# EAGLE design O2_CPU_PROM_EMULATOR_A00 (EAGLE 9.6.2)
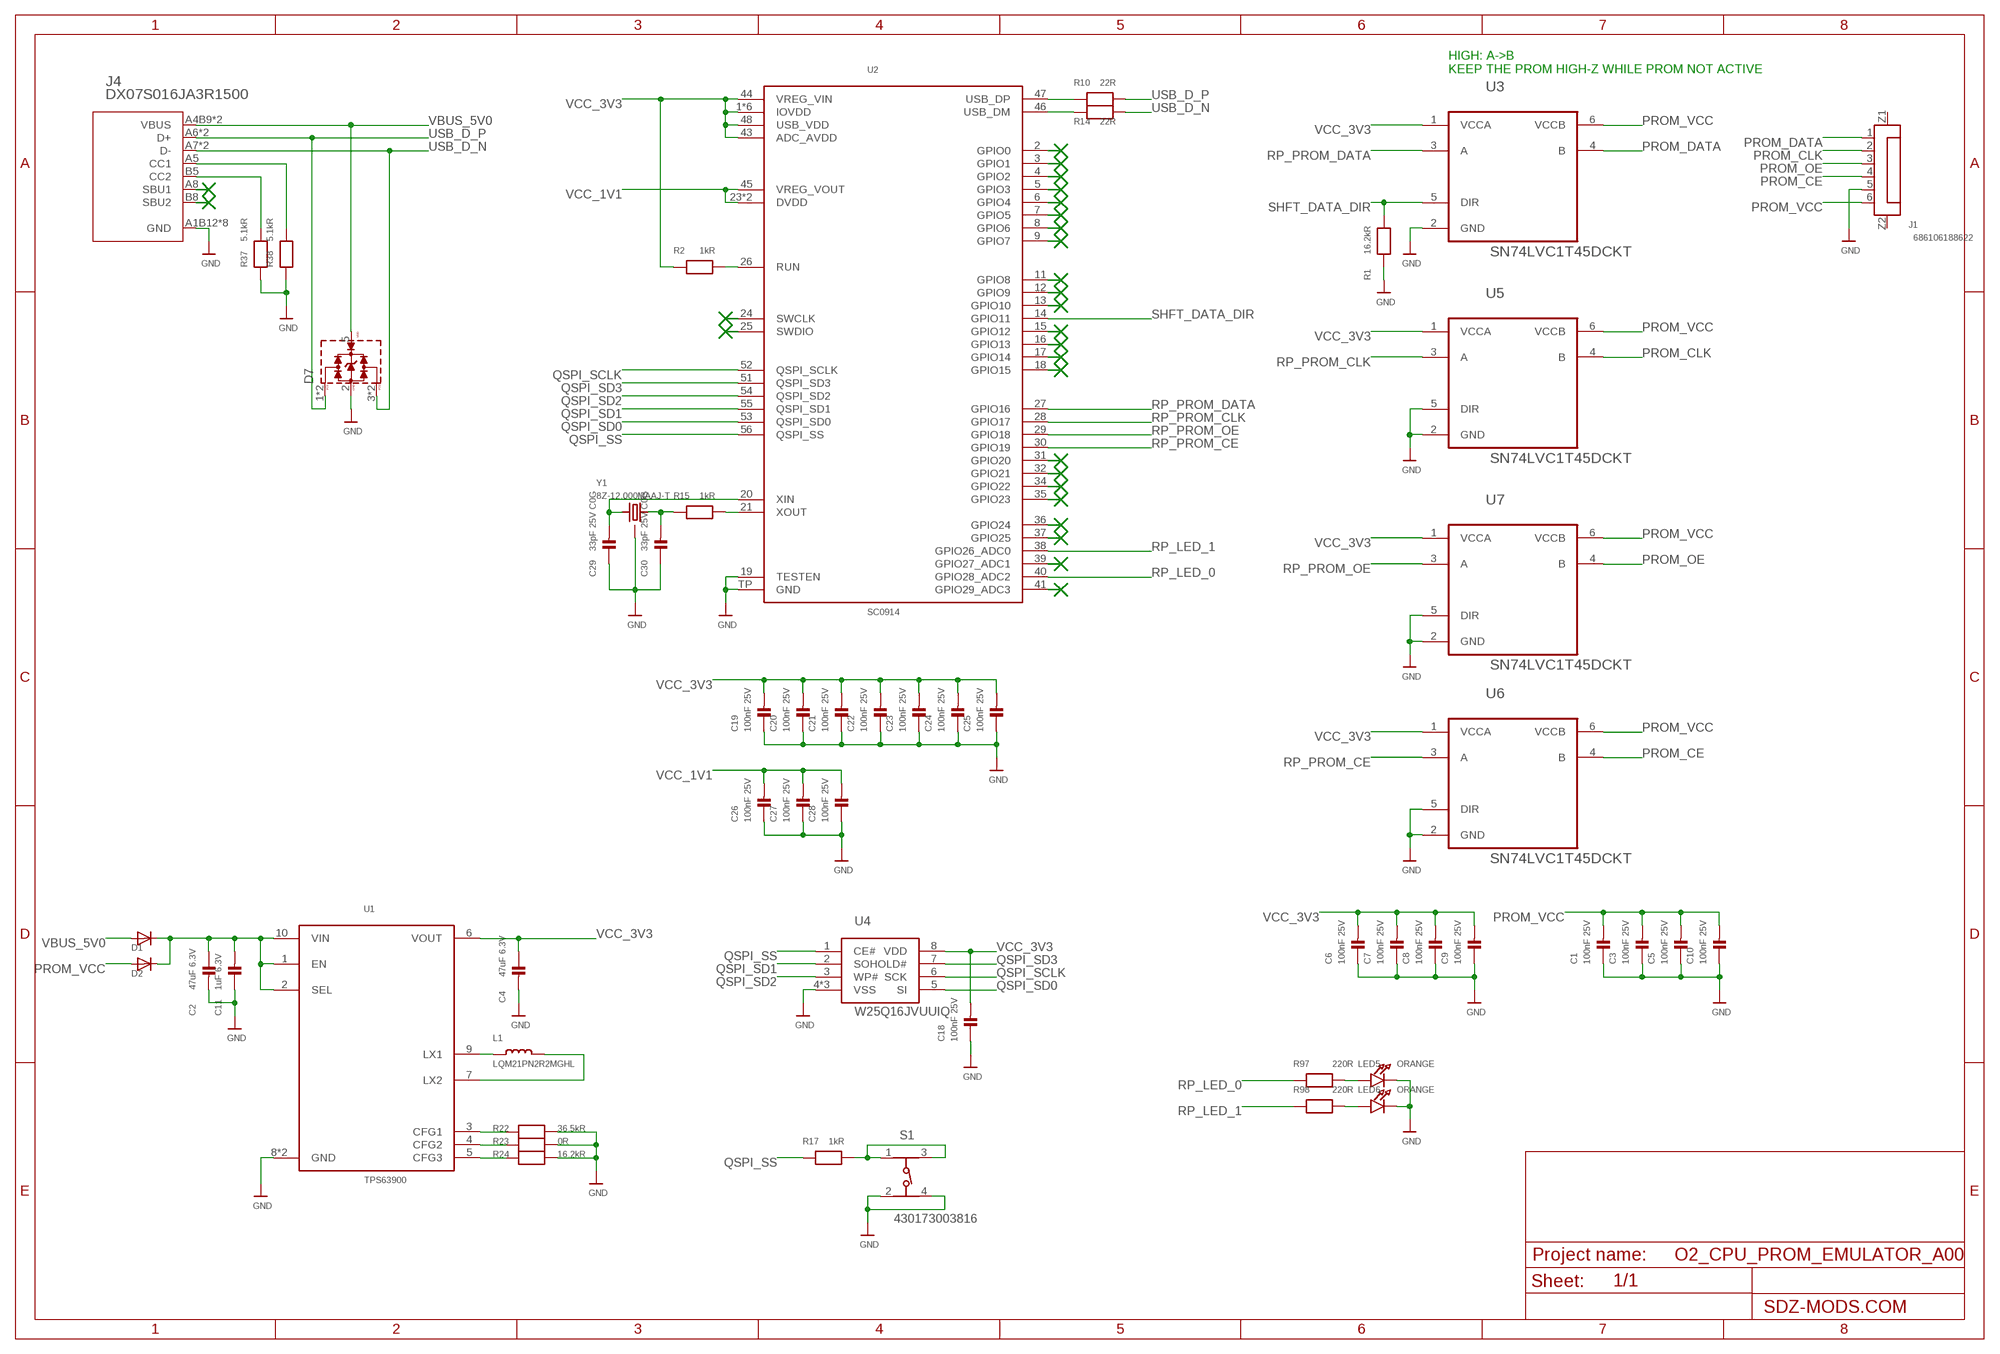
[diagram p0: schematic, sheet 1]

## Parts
C1  100nF 25V  CAP_CERAMIC0402D  [0402D]
C2  47uF 6.3V  CAP_CERAMIC0603D  [0603D]
C3  100nF 25V  CAP_CERAMIC0402D  [0402D]
C4  47uF 6.3V  CAP_CERAMIC0603D  [0603D]
C5  100nF 25V  CAP_CERAMIC0402D  [0402D]
C6  100nF 25V  CAP_CERAMIC0402D  [0402D]
C7  100nF 25V  CAP_CERAMIC0402D  [0402D]
C8  100nF 25V  CAP_CERAMIC0402D  [0402D]
C9  100nF 25V  CAP_CERAMIC0402D  [0402D]
C10  100nF 25V  CAP_CERAMIC0402D  [0402D]
C11  1uF 6.3V  CAP_CERAMIC0402D  [0402D]
C18  100nF 25V  CAP_CERAMIC0402D  [0402D]
C19  100nF 25V  CAP_CERAMIC0402D  [0402D]
C20  100nF 25V  CAP_CERAMIC0402D  [0402D]
C21  100nF 25V  CAP_CERAMIC0402D  [0402D]
C22  100nF 25V  CAP_CERAMIC0402D  [0402D]
C23  100nF 25V  CAP_CERAMIC0402D  [0402D]
C24  100nF 25V  CAP_CERAMIC0402D  [0402D]
C25  100nF 25V  CAP_CERAMIC0402D  [0402D]
C26  100nF 25V  CAP_CERAMIC0402D  [0402D]
C27  100nF 25V  CAP_CERAMIC0402D  [0402D]
C28  100nF 25V  CAP_CERAMIC0402D  [0402D]
C29  33pF 25V C0G  CAP_CERAMIC0402D  [0402D]
C30  33pF 25V C0G  CAP_CERAMIC0402D  [0402D]
D1  BAS3010B03WE6327HTSA1  [SOD-323-2]
D2  BAS3010B03WE6327HTSA1  [SOD-323-2]
D7  WE-TVS_82400152  [WE-TVS_SOT563]
J1  686106188622  6861XX188622_686106188622  [686106188622]
J4  DX07S016JA3R1500  [DX07S016JA3R1500]
L1  LQM21PN2R2MGHL  INDUCTOR_0805  [_0805@1]
LED5  ORANGE  LED  [CHIPLED_0402C]
LED6  ORANGE  LED  [CHIPLED_0402C]
R1  16.2kR  RESISTOR0402D  [0402D]
R2  1kR  RESISTOR0402D  [0402D]
R10  22R  RESISTOR0402D  [0402D]
R14  22R  RESISTOR0402D  [0402D]
R15  1kR  RESISTOR0402D  [0402D]
R17  1kR  RESISTOR0402D  [0402D]
R22  36.5kR  RESISTOR0402D  [0402D]
R23  0R  RESISTOR0402D  [0402D]
R24  16.2kR  RESISTOR0402D  [0402D]
R37  5.1kR  RESISTOR0402D  [0402D]
R38  5.1kR  RESISTOR0402D  [0402D]
R97  220R  RESISTOR0402D  [0402D]
R98  220R  RESISTOR0402D  [0402D]
S1  430173003816  [430173003816]
U1  TPS63900  [WSON10]
U2  SC0914  [QFN-56]
U3  SN74LVC1T45DCKT  [DCK]
U4  W25Q16JVUUIQ  [USON8-4X3]
U5  SN74LVC1T45DCKT  [DCK]
U6  SN74LVC1T45DCKT  [DCK]
U7  SN74LVC1T45DCKT  [DCK]
Y1  8Z-12.000MAAJ-T  TXC-8Z-25X20  [TXC-8Z-25X20]

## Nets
GND: C1.3 C2.2 C3.3 C4.2 C5.3 C6.3 C7.3 C8.3 C9.3 C10.3 C11.3 C18.3 C19.3 C20.3 C21.3 C22.3 C23.3 C24.3 C25.3 C26.3 C27.3 C28.3 C29.3 C30.3 D7.2(GND) J1.5 J4.A1B12(GND) J4.A12/B1(GND) J4.MH1(GND) J4.MH2(GND) J4.MH3(GND) J4.MH4(GND) J4.MP1(GND) J4.MP2(GND) LED5.4(C) LED6.4(C) R1.4 R22.3 R23.3 R24.3 R37.3 R38.3 S1.2 S1.4 U1.8(GND) U1.EP(GND) U2.19(TESTEN) U2.TP(GND) U3.2(GND) U4.4(VSS) U4.9(VSS) U4.10(VSS) U5.2(GND) U5.5(DIR) U6.2(GND) U6.5(DIR) U7.2(GND) U7.5(DIR) Y1.2(GND) Y1.4(GND)
N$1: J4.A5(CC1) R38.4
N$2: R22.4 U1.3(CFG1)
N$3: J4.B5(CC2) R37.4
N$4: LED5.3(A) R97.3
N$5: LED6.3(A) R98.3
N$6: R2.4 U2.26(RUN)
N$15: R10.3 U2.47(USB_DP)
N$24: R14.3 U2.46(USB_DM)
N$26: C30.4 R15.3 Y1.3
N$27: C29.4 U2.20(XIN) Y1.1
N$29: R17.4 S1.1 S1.3
N$31: R15.4 U2.21(XOUT)
N$48: R23.4 U1.4(CFG2)
N$49: R24.4 U1.5(CFG3)
N$50: L1.1 U1.9(LX1)
N$51: L1.2 U1.7(LX2)
PROM_CE: J1.4 U6.4(B)
PROM_CLK: J1.2 U5.4(B)
PROM_DATA: J1.1 U3.4(B)
PROM_OE: J1.3 U7.4(B)
PROM_VCC: C1.4 C3.4 C5.4 C10.4 D2.A J1.6 U3.6(VCCB) U5.6(VCCB) U6.6(VCCB) U7.6(VCCB)
QSPI_SCLK: U2.52(QSPI_SCLK) U4.6(SCK)
QSPI_SD0: U2.53(QSPI_SD0) U4.5(SI)
QSPI_SD1: U2.55(QSPI_SD1) U4.2(SO)
QSPI_SD2: U2.54(QSPI_SD2) U4.3(WP#)
QSPI_SD3: U2.51(QSPI_SD3) U4.7(HOLD#)
QSPI_SS: R17.3 U2.56(QSPI_SS) U4.1(CE#)
RP_LED_0: R97.4 U2.40(GPIO28_ADC2)
RP_LED_1: R98.4 U2.38(GPIO26_ADC0)
RP_PROM_CE: U2.30(GPIO19) U6.3(A)
RP_PROM_CLK: U2.28(GPIO17) U5.3(A)
RP_PROM_DATA: U2.27(GPIO16) U3.3(A)
RP_PROM_OE: U2.29(GPIO18) U7.3(A)
SHFT_DATA_DIR: R1.3 U2.14(GPIO11) U3.5(DIR)
USB_D_N: D7.3(I/O2) D7.4(I/O2) J4.A7(D-) J4.B7(D-) R14.4
USB_D_P: D7.1(I/O1) D7.6(I/O1) J4.A6(D+) J4.B6(D+) R10.4
VBUS_5V0: D1.A D7.5(VDD) J4.A4B9(VBUS) J4.B4A9(VBUS)
VCC_1V1: C26.4 C27.4 C28.4 U2.23(DVDD) U2.45(VREG_VOUT) U2.50(DVDD)
VCC_3V3: C4.1 C6.4 C7.4 C8.4 C9.4 C18.4 C19.4 C20.4 C21.4 C22.4 C23.4 C24.4 C25.4 R2.3 U1.6(VOUT) U2.1(IOVDD) U2.10(IOVDD) U2.22(IOVDD) U2.33(IOVDD) U2.42(IOVDD) U2.43(ADC_AVDD) U2.44(VREG_VIN) U2.48(USB_VDD) U2.49(IOVDD) U3.1(VCCA) U4.8(VDD) U5.1(VCCA) U6.1(VCCA) U7.1(VCCA)
VMAIN: C2.1 C11.4 D1.C D2.C U1.1(EN) U1.2(SEL) U1.10(VIN)
Unconnected: J1.Z1 J1.Z2 J4.A8(SBU1) J4.B8(SBU2) U2.2(GPIO0) U2.3(GPIO1) U2.4(GPIO2) U2.5(GPIO3) U2.6(GPIO4) U2.7(GPIO5) U2.8(GPIO6) U2.9(GPIO7) U2.11(GPIO8) U2.12(GPIO9) U2.13(GPIO10) U2.15(GPIO12) U2.16(GPIO13) U2.17(GPIO14) U2.18(GPIO15) U2.24(SWCLK) U2.25(SWDIO) U2.31(GPIO20) U2.32(GPIO21) U2.34(GPIO22) U2.35(GPIO23) U2.36(GPIO24) U2.37(GPIO25) U2.39(GPIO27_ADC1) U2.41(GPIO29_ADC3)

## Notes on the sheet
- HIGH: A->B
  KEEP THE PROM HIGH-Z WHILE PROM NOT ACTIVE

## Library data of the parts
C1-C11 C18-C30 = microbuilder:CAP_CERAMIC: Ceramic Capacitors
D1 D2 = BAS3010:BAS3010
D7 = SignalCommunications (rev18d):WE-TVS_82400152: TVS Diode High Speed Series Characteristics Low clamping voltage Sturdy design Very low capacitance Flow Thru Design for a simple layout Rail to Rail protection Epoxy flame resistant UL94 V-0 RoHS, REACH and free of halogens Applications Very fast data lines USB 2.0 Ethernet PoE VGA Sim Cards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
J1 = Eagle_WR-FPC (rev24a):6861XX188622_686106188622: WR-FPC 1.00 mm SMT LIF Horizontal Top Contact KIND PROPERTIES Pitch 1 mm MATERIAL PROPERTIES Insulator Material LCP Contact Material Phosphor Bronze Contact Plating 2.032µm Tin over 1.27µm Nickel Contact Type Stamped Solder Tabs Brass Details see: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; CONTACT-RESISTANCE: 30mOhm; DATASHEET-URL: https://www.we-online.com/redexpert/spec/686106188622?ae; IR: 1A; L: 9.8mm; PACKAGING: Tape and Reel; PART-NUMBER: 686106188622; PINS: 6; PITCH: 1mm; TYPE: Horizontal; WORKING-VOLTAGE: 125V(AC)
J4 = DX07S016JA3R1500:DX07S016JA3R1500
L1 = microbuilder:INDUCTOR: Inductors
LED5 LED6 = microbuilder:LED: LED
R1 R2 R10 R14 R15 R17 R22-R24 R37 R38 R97 R98 = microbuilder:RESISTOR: Resistors
S1 = Eagle_WS-TASV (rev21c):430173003816: WS-TASV J-Bend SMT Tact Switch 3.7x3.7 mm Material Properties Cover Material : Stainless Steel Properties Frame Material LCP Frame Flammability Rating UL94 V-0 Frame Color Black Contact Material Stainless Steel Contact Plating Silver Terminal Material Copper Alloy Terminal Plating Silver VR 12 V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; DATASHEET-URL: https://www.we-online.com/catalog/datasheet/430173003816.pdf; H: 0.35mm; OPERATION-FORCE: 160g; PART-NUMBER: 430173003816; QTY: 10000
U1 = TPS63900:TPS63900
U2 = SC0914:SC0914
U3 U5-U7 = SN74LVC1T45:SN74LVC1T45DCKT
U4 = W25Q16JVUUIQ:W25Q16JVUUIQ
Y1 = TXC-8Z-25x20:TXC-8Z-25X20

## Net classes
1 USB: width 0.11 mm, drill 0.15 mm, clearance 0.13 mm

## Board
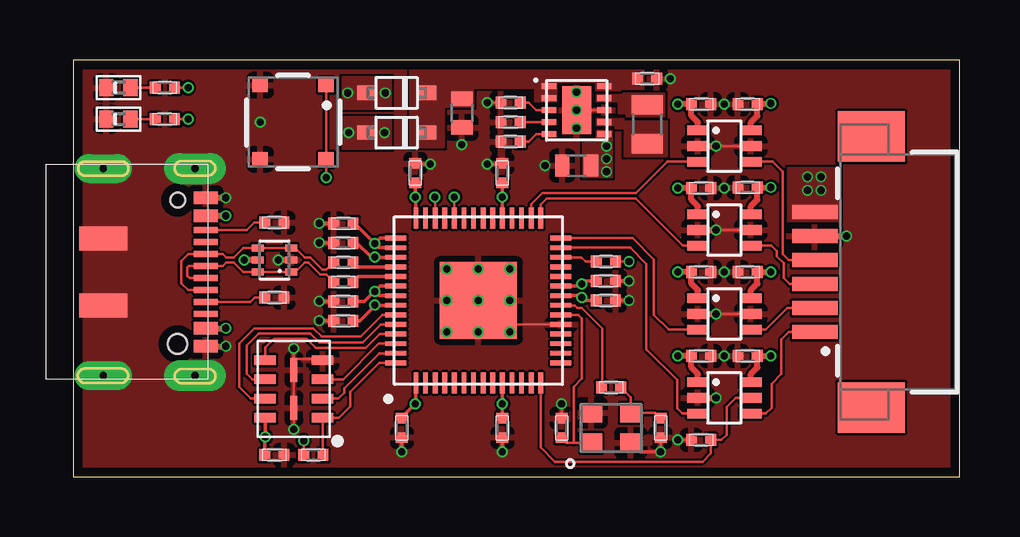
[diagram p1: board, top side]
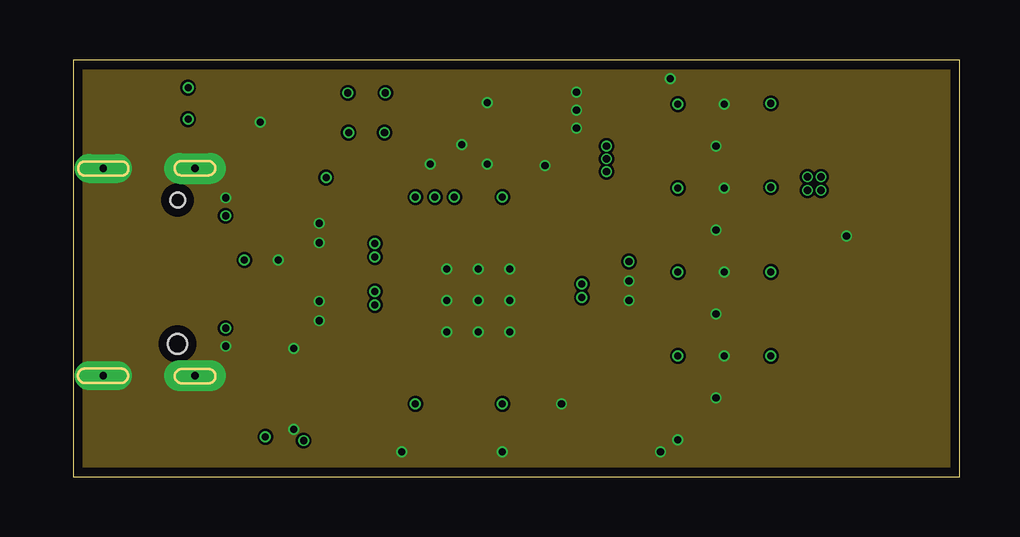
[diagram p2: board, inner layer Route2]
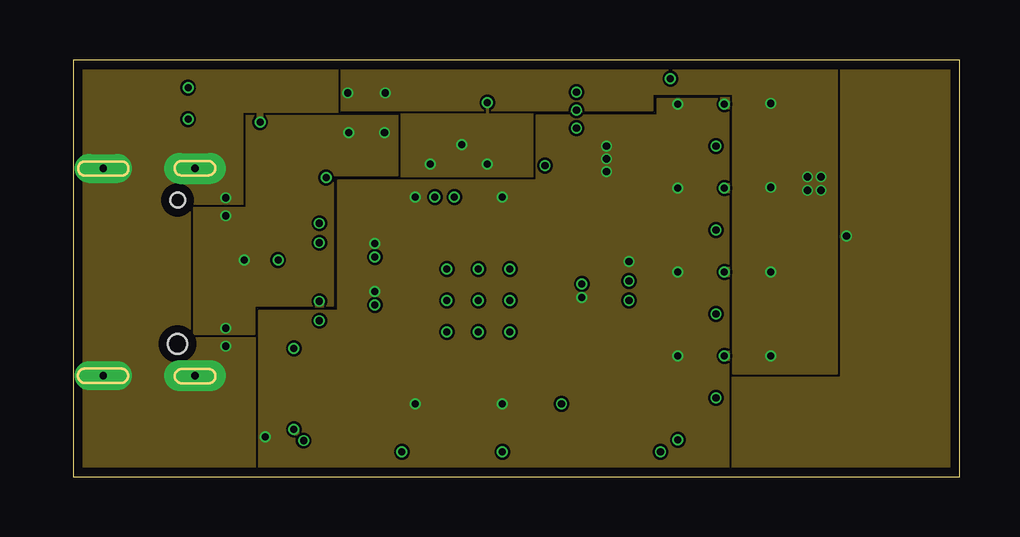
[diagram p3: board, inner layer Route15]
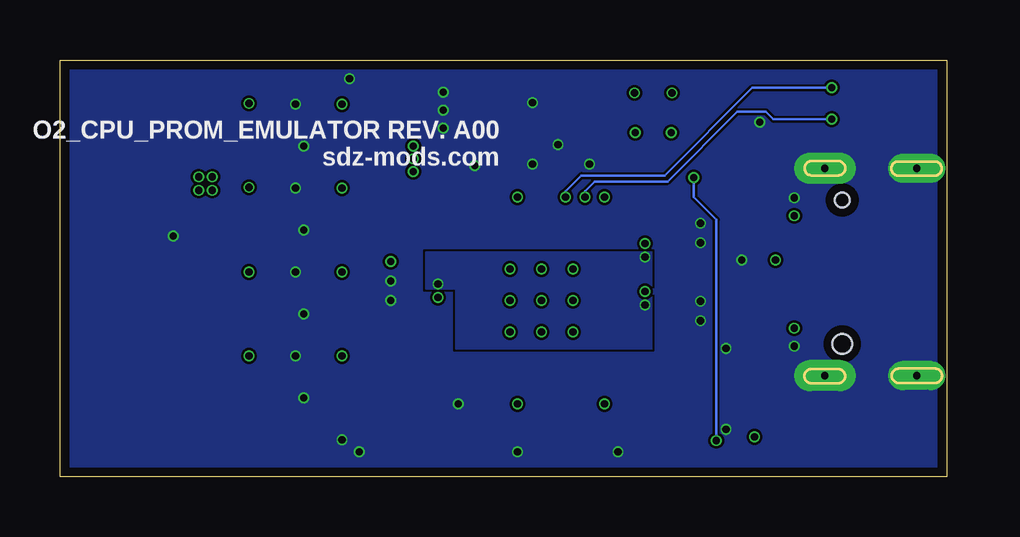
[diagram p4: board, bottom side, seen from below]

Size 36.94 x 17.38 mm. Coordinates in mm from the lower left corner, seen from the top.
Outline: 0,0 36.94,0 36.94,17.38 0,17.38 0,0
Copper layers (1+2*15+16): Top 0.035mm / dielectric 1.5mm / Route2 0.035mm / dielectric 0.15mm / Route15 0.035mm / dielectric 0.2mm / Bottom 0.035mm
Design rules "default *": minimum track width 0.1mm, minimum drill 0.3mm, track to track 0.1mm, track to pad 0.1mm, pad to pad 0.1mm, via to via 0.1mm, smd to smd 0.1mm, copper to edge 15mil, drill to drill 6mil, minimum pad ring 10mil, minimum via ring 0.075mm, stop-mask expansion 4mil, vias tented up to drill 0.4mm, thermal gap 10mil

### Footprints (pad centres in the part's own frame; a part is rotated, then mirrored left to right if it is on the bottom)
0402D = smd 0.45 x 0.5: 3 -0.403,0; 4 0.404,0
0603D = smd 0.6 x 0.9: 1 -0.6,0; 2 0.6,0
SOD-323-2 = smd 0.8 x 0.6: A -1.25,0; C 1.25,0
WE-TVS_SOT563 = smd 0.5 x 0.3: 1 -0.7,0.5; 2 -0.7,0; 3 -0.7,-0.5; 4 0.7,-0.5; 5 0.7,0; 6 0.7,0.5
686106188622 = smd 0.6 x 1.9: 1 -2.5,2.95; 2 -1.5,2.95; 3 -0.5,2.95; 4 0.5,2.95; 5 1.5,2.95; 6 2.5,2.95 | smd 2.1 x 2.8: Z1 -5.65,0.6; Z2 5.65,0.6
DX07S016JA3R1500 = smd 0.52 x 1: A1B12 -3.1,3.546; A4B9 -2.35,3.546; A12/B1 3.1,3.546; B4A9 2.35,3.546 | smd 0.27 x 1: A5 -1.75,3.55; A6 -0.25,3.55; A7 0.75,3.55; A8 1.75,3.55; B5 1.25,3.55; B6 0.25,3.55; B7 -0.75,3.55; B8 -1.25,3.55 | drill 0.3 pad 1.3 long: MH1 -4.32,3.1; MH2 4.32,3.1 | drill 0.3 pad 1.2 long: MH3 -4.32,-0.725; MH4 4.32,-0.725 | smd 1 x 2: MP1 -1.4,-0.725; MP2 1.4,-0.725 | hole 0.6: -3,2.375 | hole 0.8: 3,2.375
_0805@1 = smd 0.8 x 1.3: 1 -0.816,0; 2 0.816,0
CHIPLED_0402C = smd 0.6 x 0.7: 3 -0.502,0; 4 0.504,0
430173003816 = smd 0.6 x 0.65: 1 -1.55,1.375; 2 -1.55,-1.375; 3 1.55,1.375; 4 1.55,-1.375
WSON10 = smd 0.6 x 0.25: 1 -1.15,1; 2 -1.15,0.5; 3 -1.15,0; 4 -1.15,-0.5; 5 -1.15,-1; 6 1.15,-1; 7 1.15,-0.5; 8 1.15,0; 9 1.15,0.5; 10 1.15,1 | smd 1.2 x 2: EP 0,0
QFN-56 = smd 0.875 x 0.2: 1 -3.438,2.6; 2 -3.438,2.2; 3 -3.438,1.8; 4 -3.438,1.4; 5 -3.438,1; 6 -3.438,0.6; 7 -3.438,0.2; 8 -3.438,-0.2; 9 -3.438,-0.6; 10 -3.438,-1; 11 -3.438,-1.4; 12 -3.438,-1.8; 13 -3.438,-2.2; 14 -3.438,-2.6; 29 3.438,-2.6; 30 3.438,-2.2; 31 3.438,-1.8; 32 3.438,-1.4; 33 3.438,-1; 34 3.438,-0.6; 35 3.438,-0.2; 36 3.438,0.2; 37 3.438,0.6; 38 3.438,1; 39 3.438,1.4; 40 3.438,1.8; 41 3.438,2.2; 42 3.438,2.6 | smd 0.2 x 0.875: 15 -2.6,-3.438; 16 -2.2,-3.438; 17 -1.8,-3.438; 18 -1.4,-3.438; 19 -1,-3.438; 20 -0.6,-3.438; 21 -0.2,-3.438; 22 0.2,-3.438; 23 0.6,-3.438; 24 1,-3.438; 25 1.4,-3.438; 26 1.8,-3.438; 27 2.2,-3.438; 28 2.6,-3.438; 43 2.6,3.438; 44 2.2,3.438; 45 1.8,3.438; 46 1.4,3.438; 47 1,3.438; 48 0.6,3.438; 49 0.2,3.438; 50 -0.2,3.438; 51 -0.6,3.438; 52 -1,3.438; 53 -1.4,3.438; 54 -1.8,3.438; 55 -2.2,3.438; 56 -2.6,3.438 | smd 3.2 x 3.2: TP 0,0
DCK = smd 0.9 x 0.4: 1 -1.1,0.65; 2 -1.1,0; 3 -1.1,-0.65; 4 1.1,-0.65; 5 1.1,0; 6 1.1,0.65
USON8-4X3 = smd 0.9 x 0.4: 1 -1.2,1.2; 2 -1.2,0.4; 3 -1.2,-0.4; 4 -1.2,-1.2; 5 1.2,-1.2; 6 1.2,-0.4; 7 1.2,0.4; 8 1.2,1.2 | smd 0.3 x 1: 9 0,0.8; 10 0,-0.8
TXC-8Z-25X20 = smd 0.9 x 0.8: 1 -0.825,-0.625; 2 0.825,-0.625; 3 0.825,0.625; 4 -0.825,0.625

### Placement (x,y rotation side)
C1  28.09,5.03 0 top
C2  16.19,15.16 270 top
C3  28.09,8.53 0 top
C4  20.97,12.97 180 top
C5  28.09,12.06 0 top
C6  26.16,5.03 180 top
C7  26.16,8.53 180 top
C8  26.16,12.03 180 top
C9  26.16,15.53 180 top
C10  28.09,15.53 0 top
C11  23.91,16.59 180 top
C18  8.38,0.91 180 top
C19  11.25,7.31 0 top
C20  11.25,10.56 0 top
C21  14.25,12.66 270 top
C22  17.88,12.66 270 top
C23  22.19,7.34 180 top
C24  17.88,2.03 90 top
C25  13.69,2.03 90 top
C26  22.19,8.16 180 top
C27  11.25,6.5 0 top
C28  11.25,9.75 0 top
C29  20.34,2.03 270 top
C30  24.47,2.03 90 top
D1  13.47,14.34 0 top
D2  13.47,16 0 top
D7  8.38,9.03 180 top
J1  33.84,8.53 90 top
J4  1.97,8.53 270 top
L1  23.91,14.69 270 top
LED5  1.88,14.91 180 top
LED6  1.88,16.22 180 top
R1  26.16,1.53 180 top
R2  22.19,8.97 180 top
R10  11.25,8.12 180 top
R14  11.25,8.94 180 top
R15  22.41,3.72 180 top
R17  10,0.91 180 top
R22  18.22,15.59 0 top
R23  18.22,14.78 0 top
R24  18.22,13.97 0 top
R37  8.38,7.47 180 top
R38  8.38,10.59 180 top
R97  3.81,14.91 0 top
R98  3.81,16.22 0 top
S1  9.16,14.78 270 top
U1  20.97,15.28 0 top
U2  16.88,7.34 90 top
U3  27.12,3.28 0 top
U4  9.19,3.66 180 top
U5  27.12,6.78 0 top
U6  27.12,13.78 0 top
U7  27.12,10.28 0 top
Y1  22.41,2.03 0 top

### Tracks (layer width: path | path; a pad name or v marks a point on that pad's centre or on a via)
GND  (via drill 0.3)
  Top 0.1: U6.5 v26.78,13.78 | U7.5 v26.78,10.28 | U5.5 v26.78,6.78 | R1.4 v25.19,1.53 | R22.3 v17.25,15.59 | U1.8 U1.EP
  Top 0.102: 9.19,4.91 U4.10 U4.9 v9.19,1.97 | 9.19,4.91 v9.19,5.34 | U4.4 10.34,4.91 9.19,4.91 | U2.19 18.5,6.34 v18.19,6.03 | C29.3 v20.34,3.03 | C30.3 v24.47,1.03
  Top 0.15: v10.25,6.5 C27.3 | v10.25,7.31 C19.3 | v10.25,9.75 C28.3 | v10.25,10.56 C20.3 | C21.3 14.28,13.03 v14.88,13.03 | v17.25,13.03 17.85,13.03 C22.3 | C26.3 v23.16,8.16 | C23.3 v23.16,7.34 | C24.3 v17.88,1.03 | C25.3 v13.69,1.03 | Y1.2 23.61,1.03 v24.47,1.03 | U2.TP v16.88,6.03 | U2.TP v18.19,6.03 | U2.TP v18.19,7.34 | U2.TP v18.19,8.66 | U2.TP v16.88,8.66 | U2.TP v15.56,8.66 | U2.TP v15.56,7.34 | U2.TP v15.56,6.03
  Top 0.254: D7.2 v8.53,9.03 | J1.5 v32.22,10.03 | U6.2 v26.78,13.78 | U7.2 v26.78,10.28 | U5.2 v26.78,6.78 | U3.2 v26.78,3.28 | J4.A1B12 v6.34,11.63 | J4.A12/B1 v6.34,5.43 v6.34,5.44
  other vias: 16.88,7.34 7.78,14.78 27.12,15.53 27.12,12.03 27.12,8.53 27.12,5.03 20.97,15.28 20.97,16.03 20.97,14.53 24.88,16.59 16.19,13.84 19.66,12.97
  pour Top (rank 5): -0.44,17.78 37.47,17.78 37.47,-0.38 -0.44,-0.38
  pour Route2 (rank 5): -0.44,17.78 37.47,17.78 37.47,-0.38 -0.44,-0.38
  pour Route15 (rank 5): -0.44,17.78 37.47,17.78 37.47,-0.38 -0.44,-0.38
  pour Bottom (rank 5): -0.44,17.78 37.47,17.78 37.47,-0.38 -0.44,-0.38
N$1
  Top 0.1: J4.A5 7.22,10.28 7.53,10.59 R38.4
N$2
  Top 0.1: U1.3 19.28,15.28 18.97,15.59 R22.4
N$3
  Top 0.1: J4.B5 7.38,7.28 7.56,7.47 R37.4
N$4
  Top 0.1: LED5.3 R97.3
N$5
  Top 0.1: LED6.3 R98.3
N$6
  Top 0.1: U2.26 21.17,9.14 21.34,8.97 R2.4
N$15
  Top 0.15: U2.47 11.87,8.34 R10.3
N$24
  Top 0.15: U2.46 11.85,8.74 R14.3
N$26
  Top 0.102: C30.4 24.25,2.66 Y1.3 23.23,3.3 R15.3
N$27
  Top 0.1: 21.19,6.59 21.19,4.09 20.84,3.75 20.84,1.41
  Top 0.102: Y1.1 20.84,1.41 20.57,1.41 C29.4 | U2.20 21.04,6.74 21.19,6.59
N$29  (via drill 0.3)
  Top 0.1: R17.4 v9.6,1.5 v9.59,1.5
  Top 0.102: v10.53,12.47 S1.3 S1.1
  Bottom 0.1: v9.59,1.5 9.59,10.72 10.53,11.66 v10.53,12.47
N$31
  Top 0.1: 21.19,7.03 22.04,6.18 22.04,3.76 R15.4
  Top 0.102: U2.21 20.89,7.14 21,7.03 21.19,7.03
N$48
  Top 0.1: U1.4 R23.4
N$49
  Top 0.1: U1.5 19.28,14.28 18.97,13.97 R24.4
N$50
  pour Top (no thermals): 21.81,15.91 22.91,15.91 22.91,15.97 24.62,15.97 24.62,15.03 23.06,15.03 23.06,15.16 22.72,15.16 22.72,15.66 21.81,15.66
N$51
  pour Top (no thermals): 21.81,14.91 22.91,14.91 22.91,14.81 24.72,14.81 24.72,13.38 22.97,13.38 22.97,14.53 22.59,14.53 22.59,14.66 21.81,14.66
PROM_CE
  Top 0.1: J1.4 29.81,9.03 29.56,9.28 29.56,12.72 29.15,13.13 U6.4
PROM_CLK
  Top 0.1: J1.2 29.75,7.03 28.85,6.13 U5.4
PROM_DATA
  Top 0.1: J1.1 29.81,6.03 29.5,5.72 29.5,4.28 29.09,3.88 29.09,2.88 28.85,2.63 U3.4
PROM_OE
  Top 0.1: J1.3 29.84,8.03 29.59,8.28 29.59,8.91 29.31,9.19 29.31,9.41 29.09,9.63 U7.4
PROM_VCC  (via drill 0.3)
  Top 0.254: U3.6 28.23,4.28 28.5,4.55 C1.4 v29.06,5.03 | U5.6 28.23,7.78 28.5,8.05 C3.4 v29.06,8.53 | U7.6 28.23,11.28 28.5,11.55 C5.4 v29.06,12.06 | U6.6 28.23,14.78 28.5,15.05 C10.4 28.53,15.56 v29.06,15.56
  other vias: 31.16,11.94 30.59,11.94 30.59,12.5 31.16,12.5 13,16 11.44,16
  pour Top (no thermals): 29.78,10.66 31.94,10.66 31.94,12.88 29.78,12.88
  pour Top (no thermals): 11.22,16.66 13.22,16.66 13.22,15.34 11.22,15.34
  pour Route15: 27.5,4.31 31.81,4.31 31.81,17.22 11.19,17.22 11.19,15.28 24.12,15.28 24.12,15.97 27.5,15.97
QSPI_SCLK
  Top 0.1: U2.52 12.81,6.34 12.06,5.59 10.25,5.59 9.88,5.97 7.72,5.97 7.22,5.47 7.22,4.28 7.44,4.06 U4.6
QSPI_SD0
  Top 0.1: U2.53 12.76,5.94 12.19,5.38 10.09,5.38 9.72,5.75 8.34,5.75 7.99,5.39 U4.5
QSPI_SD1
  Top 0.1: U2.55 12.74,5.14 11.28,3.69 11.28,3.5 11.04,3.26 U4.2
QSPI_SD2
  Top 0.1: 13.41,5.58 U2.54 12.73,5.54 11.24,4.06 U4.3
  Top 0.102: 13.32,5.54 U2.54
QSPI_SD3
  Top 0.1: U2.51 12.87,6.74 11.97,5.84 10.34,5.84 10,6.19 7.53,6.19 6.91,5.56 6.91,3.75 7.4,3.26 U4.7
QSPI_SS
  Top 0.1: U2.56 12.74,4.74 11.53,3.53 11.53,2.94 11.05,2.46 U4.1
  Top 0.102: U2.56 13.44,4.72 | U4.1 10.39,0.92 R17.3
RP_LED_0  (via drill 0.3)
  Top 0.1: U2.40 15.07,11.64 v15.06,11.66 | R97.4 v4.78,14.91
  Bottom 0.1: v15.06,11.66 15.06,11.91 14.66,12.31 11.62,12.31 8.72,15.22 7.53,15.22 7.22,14.91 v4.78,14.91
RP_LED_1  (via drill 0.3)
  Top 0.1: U2.38 v15.88,11.66 | R98.4 v4.78,16.22
  Bottom 0.1: v15.88,11.66 15.88,11.91 15.22,12.56 11.75,12.56 8.09,16.22 v4.78,16.22
RP_PROM_CE
  Top 0.1: U6.3 24.74,13.13 23.43,11.82 19.54,11.82 19.07,11.36 U2.30
RP_PROM_CLK
  Top 0.1: U5.3 24.81,6.13 24.19,6.75 24.19,9.06 23.31,9.94 U2.28
RP_PROM_DATA
  Top 0.1: U3.3 25.37,2.63 25.16,2.84 25.16,4.03 23.88,5.31 23.88,8.88 23.21,9.54 U2.27
RP_PROM_OE
  Top 0.1: U7.3 25.4,9.63 23.44,11.59 19.73,11.59 19.48,11.34 U2.29
SHFT_DATA_DIR
  Top 0.1: U2.14 19.48,1.21 20.06,0.63 23.66,0.63 23.72,0.63 26.22,0.63 26.56,0.97 R1.3 27,1.53 27.22,1.75 27.22,2.91 27.59,3.28 U3.5
USB_D_N
  Top 0.1: J4.A7 4.78,7.78 4.5,8.06 4.5,9 4.78,9.28 J4.B7 6.22,9.28 6.37,9.13 6.69,9.13 7.09,9.53 D7.4 D7.3 9.12,9.53 9.24,9.53 9.64,9.13 9.87,9.13 10.37,8.63 10.53,8.63 10.83,8.94 R14.4
  Top 0.102: R14.4 10.96,8.94
USB_D_P
  Top 0.1: J4.B6 4.84,8.28 4.75,8.38 4.75,8.72 4.81,8.78 J4.A6 6.22,8.78 6.37,8.93 6.69,8.93 7.09,8.53 D7.6 D7.1 9.24,8.53 9.64,8.93 9.79,8.93 10.29,8.43 10.53,8.43 10.83,8.13 R10.4
VBUS_5V0  (via drill 0.3)
  Top 0.254: D7.5 v7.12,9.03 | J4.A4B9 v6.34,10.88 | J4.B4A9 v6.34,6.19
  other vias: 12.97,14.34 11.47,14.34
  pour Top (no thermals): 11.22,15 13.22,15 13.22,13.69 11.22,13.69
  pour Route15: 5.03,11.22 7.22,11.22 7.22,15.06 13.5,15.06 13.5,12.56 10.81,12.56 10.81,7.12 7.53,7.12 7.53,5.94 5.03,5.94
VCC_1V1  (via drill 0.3)
  Top 0.102: 12.57,9.14 v12.56,9.16
  Top 0.15: U2.23 21.1,7.94 v21.19,8.03 21.31,8.16 C26.4 | C28.4 11.81,9.75 12.4,9.16 v12.56,9.16 | C27.4 11.93,6.5 12.57,7.14 | U2.50 12.57,7.14 | 12.57,7.14 v12.56,7.16 | U2.45 12.57,9.14
  pour Bottom: 21.69,7.84 21.69,9.34 12.31,9.34 12.31,5.34 20.44,5.34 20.44,7.84
VCC_3V3  (via drill 0.3)
  Top 0.1: R2.3 v23.16,8.97
  Top 0.15: U2.22 21.11,7.54 v21.19,7.47 21.31,7.34 C23.4 | U2.33 v17.88,11.66 C22.4 | U2.42 14.27,11.63 v14.25,11.66 C21.4 | U2.43 12.79,9.94 v12.56,9.72 | U2.44 12.74,9.54 12.73,9.56 12.72,9.56 v12.56,9.72 | C20.4 11.72,10.56 v12.56,9.72 | C19.4 12.12,7.31 12.53,7.72 v12.56,7.72 | U2.10 v17.88,3.03 C24.4 | U2.49 12.74,7.54 12.73,7.56 12.72,7.56 v12.56,7.72 | U2.48 12.79,7.94 v12.56,7.72 | U4.8 7.99,1.67 v8,1.66 7.97,1.63 C18.4 | U2.1 14.27,3.06 v14.25,3.03 13.69,2.47 C25.4
  Top 0.254: U3.1 26.02,4.28 25.75,4.55 C6.4 v25.19,5.03 | U5.1 26.02,7.78 25.75,8.05 C7.4 v25.19,8.53 | U7.1 26.02,11.28 25.75,11.55 C8.4 v25.19,12.03 | U6.1 26.02,14.78 25.75,15.05 C9.4 v25.19,15.53
  other vias: 22.22,12.72 22.22,13.25 22.22,13.78
  pour Route15: 27.28,0.31 27.28,15.75 24.34,15.75 24.34,15.06 19.31,15.06 19.31,12.34 11.03,12.34 11.03,6.91 7.75,6.91 7.75,0.31
  pour Top (no thermals): 21.81,14.41 22.44,14.41 22.44,12.5 21.25,12.5 21.25,13.91 21.81,13.91
VMAIN
  pour Top (no thermals): 14.03,13.75 15.44,13.75 15.44,15.44 16.66,15.44 16.66,16.22 19.25,16.22 19.25,15.66 20.12,15.66 20.12,16.47 21.78,16.47 21.78,16.12 22.78,16.12 22.78,16.19 23.75,16.19 23.75,17.22 14.03,17.22

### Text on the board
bPlace: O2_CPU_PROM_EMULATOR REV. A00 / sdz-mods.com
